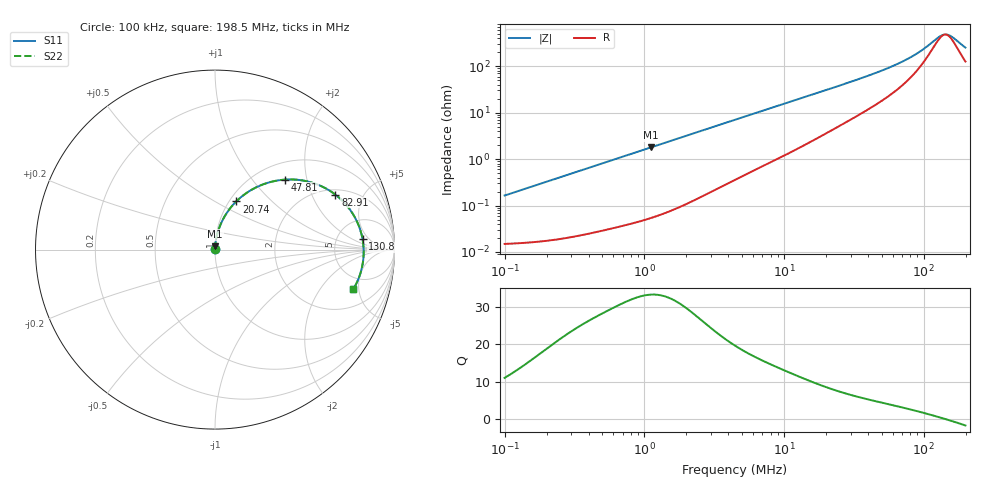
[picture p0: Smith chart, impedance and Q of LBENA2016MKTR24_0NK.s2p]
! LBENA2016MKTR24_0NK  S-PARAMETER MODEL  ( General Type )
! Model Generated by TAIYO YUDEN Corporation (http://www.ty-top.com)
! Version 1.0
! TAIYO YUDEN Control No. 211203
! Copyright(c) 2021 TAIYO YUDEN CO.,LTD. All Rights Reserved.
! Product Description (link to TY-COMPAS)
! https://ds.yuden.co.jp/TYCOMPAS/or/detail?pn=LBENA2016MKTR24M0NK&u=M
! Products Name : Inductors
! Characteristics :
!  Inductance : 0.24 uH , SRF(min) : -Hz , DC Resistance(max) : 0.018 Ohm
!  Rated Current : Saturation :6800 mA , Temp Rise : 5500 mA
!  Case Size : 2.0 x 1.6 / 0.079 x 0.063 [mm/inch] , Thickness : 1.2 / 0.047 [mm/inch]
!  (Conditions: Temperature = 25 degC , DC Bias Current/Voltage = 0A / 0V)
! External Node Assignments :
!  1  o---GGG---o  2
! GND o---------o GND
! Frequency Range : 0.1MHz  -  198.534594MHz  [ 402 STEP ]
# MHz S RI R 50
! Freq[MHz].  S11 Real  S11 Imag  S21 Real  S21 Imag  S12 Real  S12 Imag  S22 Real  S22 Imag
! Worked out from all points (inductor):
!   401 points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, 100 kHz to 198.5 MHz, reference 50 ohm
!   read as one part in series: L = 260 nH near 103.9 kHz
!   highest Q = 33.2 at 1.114 MHz (marker M1), where L = 255 nH
!   self-resonance near 142.3 MHz
!   S11 on the Smith chart (normalised r, x): 100 kHz: 1.00, +0.00; 20.74 MHz: 1.08, +0.63; 47.81 MHz: 1.33, +1.49; 82.91 MHz: 2.25, +3.03; 130.8 MHz: 9.17, +3.31; 198.5 MHz: 3.52, -4.35
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0.1  0.000152 0.00164  0.9998 -0.00164  0.9998 -0.00164  0.000152 0.00164
0.356769  0.000264 0.0058  0.9997 -0.0058  0.9997 -0.0058  0.000264 0.0058
1.114456  0.000857 0.0179  0.9991 -0.0179  0.9991 -0.0179  0.000857 0.0179
1.272844  0.00103 0.0204  0.999 -0.0204  0.999 -0.0204  0.00103 0.0204
4.541117  0.0087 0.0706  0.9913 -0.0706  0.9913 -0.0706  0.0087 0.0706
8.65922  0.0266 0.1293  0.9734 -0.1293  0.9734 -0.1293  0.0266 0.1293
15.89665  0.0759 0.2191  0.9241 -0.2191  0.9241 -0.2191  0.0759 0.2191
20.73624  0.1181 0.2681  0.8819 -0.2681  0.8819 -0.2681  0.1181 0.2681
31.48552  0.2246 0.3445  0.7754 -0.3445  0.7754 -0.3445  0.2246 0.3445
38.79729  0.3 0.3741  0.7 -0.3741  0.7 -0.3741  0.3 0.3741
47.80705  0.3907 0.39  0.6093 -0.39  0.6093 -0.39  0.3907 0.39
56.71438  0.4746 0.3872  0.5254 -0.3872  0.5254 -0.3872  0.4746 0.3872
68.57079  0.5736 0.3614  0.4264 -0.3614  0.4264 -0.3614  0.5736 0.3614
82.90582  0.6706 0.3065  0.3294 -0.3065  0.3294 -0.3065  0.6706 0.3065
100.2377  0.7537 0.2207  0.2463 -0.2207  0.2463 -0.2207  0.7537 0.2207
114.4835  0.7966 0.1442  0.2034 -0.1442  0.2034 -0.1442  0.7966 0.1442
130.7541  0.8222 0.0579  0.1778 -0.0579  0.1778 -0.0579  0.8222 0.0579
141.0696  0.828 0.0059  0.172 -0.0059  0.172 -0.0059  0.828 0.0059
152.199  0.827 -0.0468  0.173 0.0468  0.173 0.0468  0.827 -0.0468
161.1186  0.8217 -0.086  0.1783 0.086  0.1783 0.086  0.8217 -0.086
191.138  0.7832 -0.198  0.2168 0.198  0.2168 0.198  0.7832 -0.198
198.5346  0.7704 -0.2209  0.2296 0.2209  0.2296 0.2209  0.7704 -0.2209
